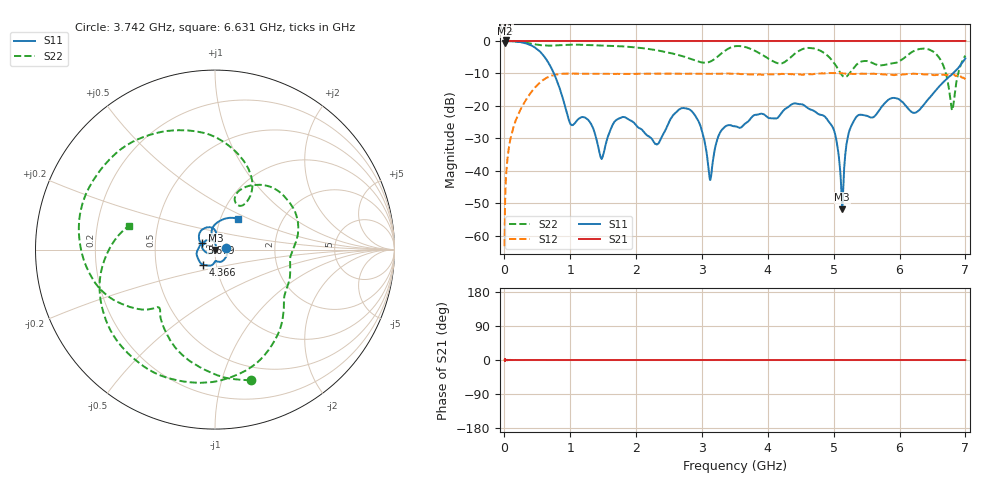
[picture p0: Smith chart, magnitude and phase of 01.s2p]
!Keysight Technologies,N5232A,MY52221221,A.10.65.11
!Date: Wednesday, October 16, 2024 11:48:51
!Correction: S11(Full 2 Port(1,4))
!S41(Full 2 Port(1,4))
!S14(Full 2 Port(1,4))
!S44(Full 2 Port(1,4))
!S2P File: Measurements: S11, S41, S14, S44:
# Hz S  RI  R 50
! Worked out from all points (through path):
!   4000 points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, 2.05 MHz to 7 GHz, reference 50 ohm
!   highest |S21| = 0.16 dB at 17.8 MHz (marker M1); lowest = -0.7 dB at 2.05 MHz (marker M2)
!   lowest |S11| = -51.8 dB at 5.129 GHz (marker M3), VSWR 1.01, Z = 50.2 - j0.146 ohm
!   |S11| at or under -10 dB: 750.7 MHz to 6.811 GHz (6.06 GHz wide, 160 % of centre)
!   |S22| runs from -21.3 to 0.0 dB; largest |S21 - S12| = 1.3
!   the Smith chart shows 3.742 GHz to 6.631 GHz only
!   S11 on the Smith chart (normalised r, x): 3.742 GHz: 1.14, +0.03; 4.366 GHz: 0.87, -0.15; 5.679 GHz: 0.86, +0.06; 6.631 GHz: 1.20, +0.44
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2049925  -0.9701 0.15  0.9176 -0.0149  0.000124 0.000684  -0.9788 0.097
1.779925e7  -0.9876 0.1518  1.019 0.00146  0.000708 0.00606  -0.9994 0.0613
1.840421e8  -0.00698 0.9766  0.9983 -0.000908  0.0619 0.0186  -0.8078 0.5538
3.415354e8  0.8927 0.1656  1 0.000451  0.0874 -0.0979  -0.4313 0.8306
4.867792e8  0.2819 -0.7091  1 -0.00043  -0.0803 -0.1879  -0.0509 0.8794
6.320229e8  -0.4585 -0.2594  0.9996 2.46e-05  -0.2685 0.0101  0.271 0.806
1.16925e9  0.0315 0.0593  1 1.42e-05  0.1625 -0.2669  0.8437 -0.2235
1.687228e9  0.0596 0.000173  0.9997 -0.000383  -0.0321 0.3098  -0.1278 -0.8276
2.3347e9  -0.00265 0.0261  0.9998 -0.000609  -0.2861 -0.1289  -0.6373 0.3218
2.80893e9  0.0785 -0.0407  0.9996 -0.000535  0.2932 0.1118  0.1085 0.5274
3.125666e9  0.0023 -0.0069  0.9997 2.42e-05  -0.059 -0.3063  0.3134 0.3655
3.5019e9  -0.048 0.00762  0.9999 -0.000347  -0.1236 0.2867  0.7906 -0.2512
3.74164e9  0.0635 0.0113  1 -0.000396  0.2829 0.1109  0.1984 -0.7269
4.366363e9  -0.065 -0.0845  1 -0.000819  -0.2433 0.1896  -0.4923 -0.3133
4.66735e9  -0.0838 0.0236  0.9993 -0.000488  0.2716 0.1433  -0.6196 0.4666
5.12933e9  0.00212 -0.00146  0.9999 4.88e-05  -0.2834 -0.1433  0.1577 0.2488
5.678807e9  -0.074 0.0362  1 -0.000532  0.3067 -0.0377  0.4238 -0.0285
5.83455e9  -0.0864 0.091  1 -8.4e-05  0.1152 -0.2791  0.4173 -0.1508
6.30703e9  -0.0172 0.0862  1 -0.000786  -0.0833 0.2992  -0.1466 -0.7385
6.630766e9  0.1264 0.1725  1 -0.000867  0.2694 -0.1236  -0.4781 0.1332
6.800509e9  0.2901 -0.106  1 -0.000619  -0.0415 -0.3071  -0.0856 -0.00444
7e9  -0.4415 -0.3109  1 -0.00158  -0.2504 0.0544  -0.5933 -0.0489
